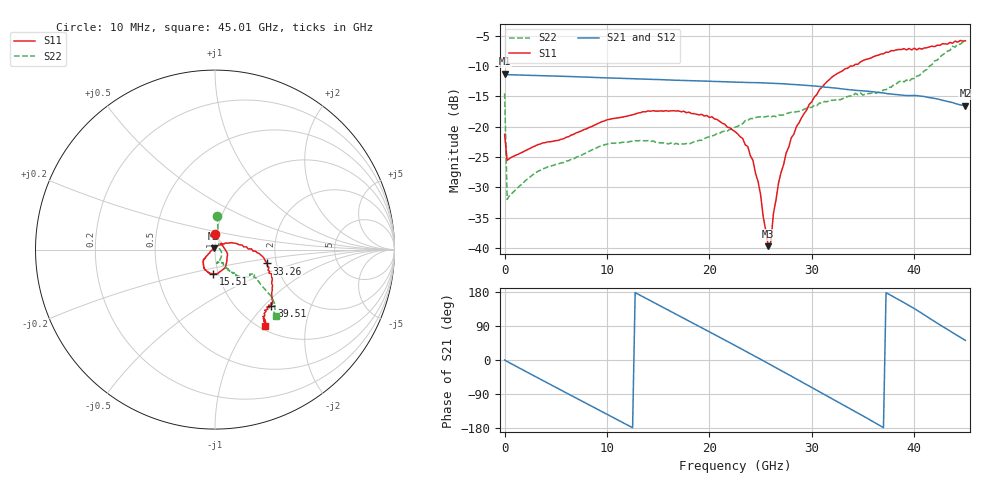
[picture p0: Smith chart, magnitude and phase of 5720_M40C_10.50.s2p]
! Device:  ADRF5720
! Description: 0.5dB LSB GaAs MMIC 6-bit Digital Attenuator
! Frequency:  0.000009 -  40 GHz
! Ports:
!	RF1	= Port 1
!	RF2	= Port 2
! Vdd:  3.3 Volt
! Vss:  -3.3 Volt
! Control:  0/3.3 Volt
! State:  10.50 dB attenuation
! Data:  The device was measured using G-S-G Probes on a matrix board.
!  Data was collected using an calibrated 4 port network analyzer.
!  The reference plane for this measurement is at the launchers.
! Note:  Analog Devices supplies this data as a sample of measured data
!  for this product.  Your particular data for this product may vary.
!  Data was taken at -40 degrees C.
!  Analog Devices reserves the right to change this data at anytime.
# GHZ S DB R 45.0
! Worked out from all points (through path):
!   181 points, 10 MHz to 45.01 GHz, reference 45 ohm
!   highest |S21| = -11.23 dB at 10 MHz (marker M1); lowest = -16.5 dB at 45.01 GHz (marker M2)
!   group delay of S21, straight-line fit = 40.8 ps
!   lowest |S11| = -39.7 dB at 25.76 GHz (marker M3), VSWR 1.02, Z = 44.4 + j0.698 ohm
!   |S11| at or under -10 dB: start of sweep to 33.75 GHz
!   |S22| runs from -32.0 to -5.9 dB; largest |S21 - S12| = 0.0011
!   S11 on the Smith chart (normalised r, x): 10 MHz: 0.99, +0.17; 15.51 GHz: 0.95, -0.26; 33.26 GHz: 1.79, -0.30; 39.51 GHz: 1.42, -1.10; 45.01 GHz: 1.05, -1.22
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0.01  -21.25 89.3  -11.23 -0.1  -11.25 -0.1  -14.48 86.4
0.26  -25.53 8.0  -11.40 -4.0  -11.42 -4.0  -31.98 16.8
4.26  -22.48 -21.0  -11.60 -61.5  -11.63 -61.5  -26.59 -33.9
7.76  -20.46 -46.4  -11.79 -111.3  -11.81 -111.3  -24.46 -60.2
11.76  -18.31 -70.9  -12.03 -168.1  -12.05 -168.1  -22.53 -77.5
15.26  -17.37 -92.6  -12.22 142.1  -12.24 142.1  -22.65 -81.8
15.51  -17.42 -94.0  -12.24 138.6  -12.26 138.5  -22.66 -81.3
19.01  -18.03 -114.5  -12.43 88.7  -12.46 88.6  -22.24 -67.0
22.76  -21.15 -138.5  -12.64 34.7  -12.66 34.6  -19.93 -60.8
24.26  -25.51 -143.3  -12.72 13.0  -12.74 12.9  -18.64 -59.9
25.01  -31.19 -159.6  -12.74 1.9  -12.76 1.8  -18.33 -58.4
25.76  -39.69 130.7  -12.81 -9.2  -12.83 -9.3  -18.24 -58.4
26.01  -38.96 96.8  -12.81 -12.8  -12.84 -13.0  -18.41 -58.5
26.26  -34.34 68.7  -12.83 -16.6  -12.85 -16.8  -18.22 -57.1
26.76  -29.29 52.2  -12.89 -24.1  -12.91 -24.2  -18.06 -57.1
27.51  -24.30 31.2  -12.93 -35.2  -12.96 -35.3  -17.83 -57.7
30.26  -15.08 4.9  -13.27 -76.6  -13.29 -76.7  -16.44 -55.0
33.26  -10.42 -14.8  -13.81 -121.5  -13.84 -121.7  -15.13 -51.7
37.76  -7.44 -40.9  -14.60 170.3  -14.63 170.1  -13.47 -46.1
39.51  -7.08 -44.8  -14.84 144.0  -14.87 143.8  -12.52 -35.3
42.26  -6.54 -54.2  -15.40 97.3  -15.42 97.1  -9.01 -38.4
45.01  -5.82 -56.7  -16.54 51.8  -16.57 51.7  -5.94 -47.5
